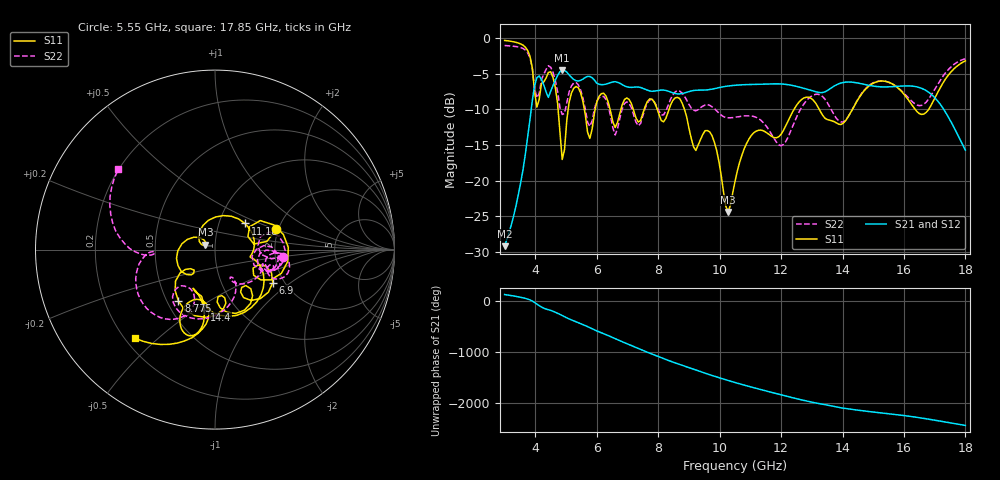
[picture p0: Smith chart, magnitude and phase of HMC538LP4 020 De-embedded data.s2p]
! Chelmsford, MA 01824
! http://www.hittite.com
! Tel: 978-250-3343
! Fax: 978-250-3373
! Device  :  HMC538LP4
! Description:  600 Analog Phase Shifter
! Frequency  :  6.0 GHz - 15.0 GHz
! Package  :  LP4  - 4x4 mm Quad Flatpack No-Lead (QFN) Plastic Package: 24 pin
! Ports  :  2 RF, 1 DC
!  Pin  3  = Rfin  = Port 1
!  Pin  16  = Rfout = Port 2
!  pin  21  = vCTL
! Voltages:  VCTL  = 0 to 5.0 Volts
! Currents :  Vb(V)  Vd(V)  Ib(mA)  Id(mA)
!  0.00  2.00  0.000000	0.474918
! Data:  The device was measured on evaluation board 111296-1.
!  Data was collected using a calibrated network analyzer.
!  The evaluation circuit board was modeled and simulated.This was use
!  to removed the evaluation board circuit from the measured data.
!  The reference plane is the center of the package pin.
! Misc:  Lot #
!Date Measured:  03 - 11 -2009
! Date:  03 - 17 -2009
! Note:
!  Hittite Microwave supplies this data as a sample of measured data at the
!  package pin for this package product.  Your particular data for this product
!  may vary.
!  Data was taken at 25 degrees C.
!  Hittite Microwave reserves the right to change this data at anytime.
# MHz S MA R 50
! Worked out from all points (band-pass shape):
!   201 points, 3 GHz to 18 GHz, reference 50 ohm
!   highest |S21| = -4.48 dB at 4.875 GHz (marker M1); lowest = -29.2 dB at 3 GHz (marker M2)
!   |S21| within 3 dB of the highest: 4.496 GHz to 8.36 GHz (3.864 GHz wide, 60.1 % of centre); 9.003 GHz to 13.11 GHz (4.106 GHz wide, 37.1 % of centre)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
!   lowest |S11| = -24.4 dB at 10.28 GHz (marker M3), VSWR 1.13, Z = 44.9 + j2.48 ohm
!   |S11| at or under -10 dB: 8.856 GHz to 12.42 GHz (3.565 GHz wide, 33.5 % of centre); 13.24 GHz to 14.32 GHz (1.077 GHz wide, 7.82 % of centre); 16.37 GHz to 16.8 GHz (436.1 MHz wide, 2.63 % of centre)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
!   |S22| runs from -15.1 to -1.0 dB; largest |S21 - S12| = 0.006
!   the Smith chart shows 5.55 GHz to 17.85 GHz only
!   S11 on the Smith chart (normalised r, x): 5.55 GHz: 1.95, +0.50; 6.9 GHz: 1.75, -0.75; 8.775 GHz: 0.57, -0.37; 11.18 GHz: 1.33, +0.41; 14.4 GHz: 0.71, -0.54; 17.85 GHz: 0.24, -0.42
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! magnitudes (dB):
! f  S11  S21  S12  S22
! 3 GHz  -0.3  -29.2  -29.2  -1.0
! 3.75 GHz  -1.7  -13.9  -13.9  -2.0
! 4.05 GHz  -9.7  -5.5  -5.5  -8.4
! 4.5 GHz  -4.7  -7.4  -7.4  -4.1
! 4.875 GHz  -17.0  -4.5  -4.5  -10.7
! 5.175 GHz  -7.7  -5.5  -5.5  -6.7
! 5.55 GHz  -8.9  -5.7  -5.7  -8.4
! 5.775 GHz  -14.1  -5.4  -5.4  -12.4
! 6.9 GHz  -8.6  -6.7  -6.7  -9.2
! 8.025 GHz  -10.7  -7.3  -7.3  -10.2
! 8.775 GHz  -9.1  -7.8  -7.8  -7.7
! 9.75 GHz  -13.7  -7.1  -7.2  -9.6
! 10.28 GHz  -24.4  -6.7  -6.7  -11.2
! 10.5 GHz  -20.1  -6.6  -6.6  -11.1
! 11.18 GHz  -13.1  -6.5  -6.5  -11.1
! 12 GHz  -13.5  -6.4  -6.4  -15.1
! 13.05 GHz  -8.7  -7.4  -7.4  -8.0
! 14.4 GHz  -9.4  -6.2  -6.2  -9.3
! 15.53 GHz  -6.2  -6.8  -6.8  -6.2
! 16.65 GHz  -10.6  -7.2  -7.2  -9.3
! 17.85 GHz  -3.5  -14.4  -14.4  -3.1
! 18 GHz  -3.2  -15.7  -15.7  -2.9
